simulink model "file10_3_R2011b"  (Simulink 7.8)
settings: Solver=ode4  StartTime=0.0  StopTime=10  FixedStep=1e-3  RelTol=1e-3

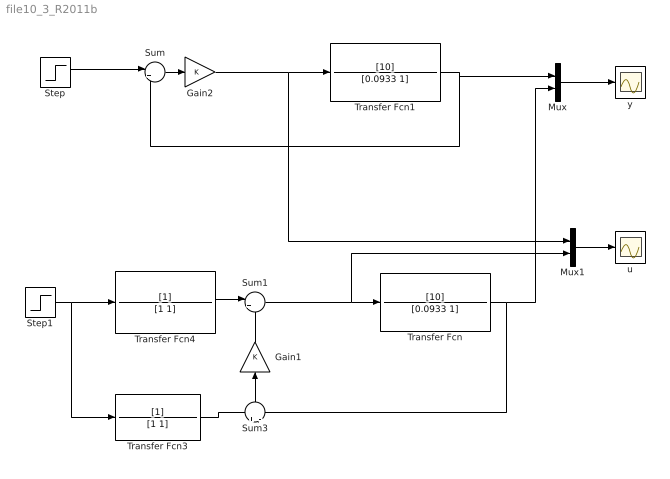
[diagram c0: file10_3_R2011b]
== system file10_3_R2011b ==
  Gain1 : Gain
  Gain2 : Gain
  Mux : Mux  Inputs=2
  Mux1 : Mux  Inputs=2
  Step : Step  SampleTime=0
  Step1 : Step  SampleTime=0
  Sum : Sum  Inputs=|+-
  Sum1 : Sum  Inputs=|++
  Sum3 : Sum  Inputs=+|-
  Transfer Fcn : TransferFcn  Numerator=[10]  Denominator=[0.0933 1]
  Transfer Fcn1 : TransferFcn  Numerator=[10]  Denominator=[0.0933 1]
  Transfer Fcn3 : TransferFcn  Denominator=[1 1]
  Transfer Fcn4 : TransferFcn  Denominator=[1 1]
  u : Scope
  y : Scope
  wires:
  Transfer Fcn1/1 -> Mux/1, Sum/2
  Sum/1 -> Gain2/1
  Transfer Fcn/1 -> Mux/2, Sum3/2
  Step1/1 -> Transfer Fcn3/1, Transfer Fcn4/1
  Transfer Fcn3/1 -> Sum3/1
  Sum3/1 -> Gain1/1
  Transfer Fcn4/1 -> Sum1/1
  Mux/1 -> y/1
  Mux1/1 -> u/1
  Step/1 -> Sum/1
  Gain1/1 -> Sum1/2
  Gain2/1 -> Transfer Fcn1/1, Mux1/1
  Sum1/1 -> Mux1/2, Transfer Fcn/1
